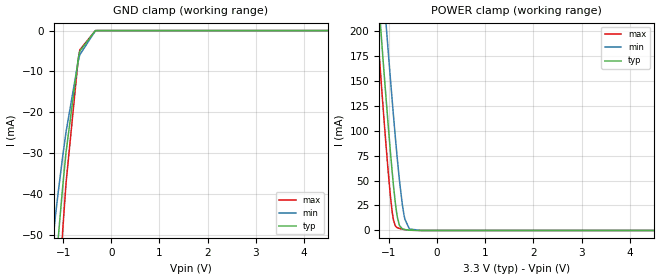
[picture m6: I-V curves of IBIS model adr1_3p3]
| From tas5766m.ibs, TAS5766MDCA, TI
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|   adr1_3p3 Model
[Model]   adr1_3p3
Model_type   Input
Vinl = 0.8
Vinh = 2
|   typ   min   max
|   (nom PVT)   (fast PVT)   (slow PVT)
C_comp   6.403e-12   6.276e-12   6.468e-12
| Where nom  PVT is Nominal Process, 3.3V, 27C
|   Fast PVT is Strong Process,  3.6V, -40C
|   Slow PVT is Weak Process,   3V, 125C
[Voltage Range]   3.3   3   3.6
|Junction Temperature
[Temperature Range]   27   125   -40
[Power Clamp Reference]   3.3   3   3.6
[GND Clamp Reference]   0   0   0
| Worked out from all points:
|   POWER clamp passes 1 mA (typ) near -0.68 V on its own axis
[GND Clamp]
|   Voltage   I(typ)   I(min)   I(max)
-3.3V     -1.485A    -1.2A      -1.772A
-1.386V   -96.7mA    -70.76mA   -130.7mA
-1.158V   -58.92mA   -45.18mA   -77.81mA
-1.109V   -51.69mA   -40.2mA    -67.73mA
-1.01V    -38.27mA   -30.85mA   -49.07mA
-940.5mV  -29.83mA   -24.85mA   -37.43mA
-687mV    -6.913mA   -7.53mA    -6.991mA
-654mV    -5.033mA   -5.917mA   -4.726mA
-330mV    -3.926uA   -36.38uA   -391.7nA
6.6V      0A         0A         0A
[POWER Clamp]
|   Voltage   I(typ)   I(min)   I(max)
-3.3V     1.681A     1.717A     1.676A
-1.27V    266.2mA    339.1mA    220.3mA
-1.136V   179.5mA    253.7mA    132.2mA
-1.08V    144.2mA    218.5mA    96.67mA
-1.018V   106.3mA    180.3mA    59.64mA
-934.8mV  59.44mA    131.1mA    19.28mA
-902.4mV  43.04mA    112.6mA    9.674mA
-825mV    13.11mA    70.88mA    2.758mA
-778.8mV  4.734mA    48.61mA    1.969mA
-690mV    1.091mA    16.09mA    1mA
-576mV    305.7uA    1.518mA    242.8uA
6.6V      0A         0A         0A
